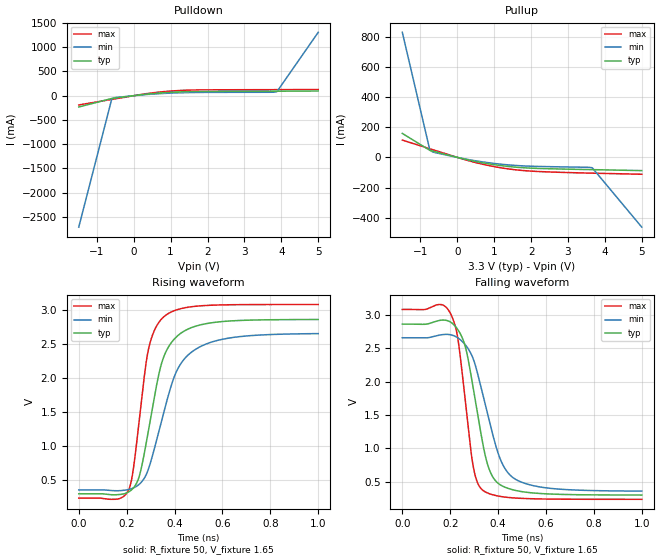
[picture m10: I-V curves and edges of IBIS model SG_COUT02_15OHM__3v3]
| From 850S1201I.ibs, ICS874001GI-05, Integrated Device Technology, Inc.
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[Model] SG_COUT02_15OHM__3v3
Model_type   Output
Polarity   Non-Inverting
|   typ   min   max
C_comp   2pF   1.5pF   2.5pF
Vmeas = 1.65V
Rref = 50
Cref = 0
Vref = 1.65V
|   typ   min   max
[Voltage range]   3.3V   3.135V   3.465V
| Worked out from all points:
|   slope of the pulldown table from 0 to 0.495 V, typ, clamps not added: 11.8 ohm
|   slope of the pullup table from 0 to 0.495 V, typ, clamps not added: 18.2 ohm
|   rising waveform, R_fixture 50, V_fixture 1.65: 20-80 % time 89.8ps typ, 119ps min, 63.9ps max; typ from 0.298 V to 2.86 V
|   falling waveform, R_fixture 50, V_fixture 1.65: 20-80 % time 77.7ps typ, 103ps min, 55.3ps max; typ from 2.86 V to 0.298 V
[Pulldown]
|Voltage   I (typ)   I (min)   I (max)
-1.49V    -233.4mA   -2.715A    -191mA
-594.8mV  -57.56mA   -66.07mA   -76.46mA
-520.2mV  -49.98mA   -41.08mA   -67.24mA
151.1mV   14.45mA    11.1mA     19.95mA
1.196V    77.02mA    59.07mA    105.5mA
3.881V    92.75mA    83.31mA    124.8mA
5V        96.89mA    1.309A     128.2mA
[Pullup]
|Voltage   I (typ)   I (min)   I (max)
-1.49V    158.8mA    828.9mA    114.5mA
-744mV    46.58mA    48.48mA    56.94mA
-594.8mV  36.89mA    31.23mA    45.73mA
151.1mV   -8.979mA   -7.489mA   -11.29mA
673.3mV   -35.45mA   -29.46mA   -44.73mA
1.27V     -57.12mA   -47.25mA   -72.38mA
2.091V    -72.31mA   -59.29mA   -92.33mA
3.657V    -81.16mA   -68.9mA    -104.6mA
5V        -87.71mA   -462.4mA   -111.8mA
[Ramp]
|   typ   min   max
dV/dt_r   2.064/0.155n   1.85/0.206n   2.294/0.109n
dV/dt_f   2.101/0.129n   1.882/0.173n   2.339/0.091n
R_load =   50.0000
[Rising Waveform]
R_fixture = 50
V_fixture = 1.65   |Vcc_typ
V_fixture_min = 1.5675 |Vcc_min
V_fixture_max = 1.7325 |Vcc_max
C_fixture = 0.0p
| Time   typ   min   max
0s        297.6mV    354.5mV    233.8mV
208.2ps   325.4mV    360.6mV    356mV
225.2ps   371.9mV    379.5mV    598.1mV
251.3ps   539.2mV    434.2mV    1.341V
290.3ps   1.217V     654.7mV    2.41V
333.3ps   2.04V      1.202V     2.815V
359.4ps   2.352V     1.557V     2.916V
419.4ps   2.643V     2.175V     3.017V
512.5ps   2.788V     2.473V     3.066V
1ns       2.864V     2.656V     3.085V
[Falling Waveform]
R_fixture = 50
V_fixture = 1.65   |Vcc_typ
V_fixture_min = 1.5675 |Vcc_min
V_fixture_max = 1.7325 |Vcc_max
C_fixture = 0.0p
| Time   typ   min   max
0s        2.864V     2.66V      3.085V
162.2ps   2.924V     2.704V     3.157V
207.2ps   2.88V      2.699V     2.978V
234.2ps   2.769V     2.652V     2.594V
264.3ps   2.512V     2.549V     1.672V
295.3ps   1.923V     2.351V     744.5mV
336.3ps   1.065V     1.804V     369.1mV
407.4ps   455.3mV    853.2mV    278.3mV
472.5ps   367.5mV    534.9mV    253.1mV
1ns       298.1mV    356.8mV    233.9mV
